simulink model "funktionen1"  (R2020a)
settings: Solver=ode45  StartTime=0.0  StopTime=10.0  MaxStep=1e-2  RelTol=1e-3  EnableMultiTasking=on
libraries: simulink x1

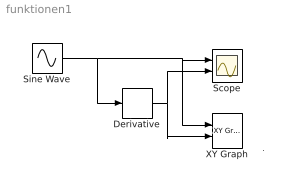
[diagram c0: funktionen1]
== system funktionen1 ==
  note: .
  Derivative : Derivative
  Scope : Scope  NumInputPorts=2
  Sine Wave : Sin  Amplitude=2  Frequency=4  Phase=-1  SampleTime=0
  XY Graph : simulink/Sinks/XY Graph  xmin=-2.2  xmax=2.2  ymin=-9  ymax=9  st=-1
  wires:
  Derivative/1 -> Scope/2, XY Graph/2
  Sine Wave/1 -> Derivative/1, Scope/1, XY Graph/1
